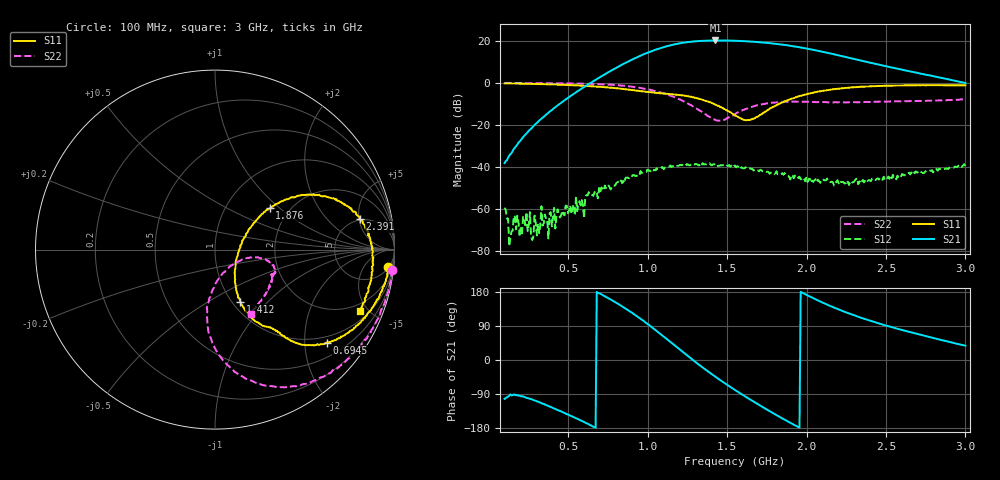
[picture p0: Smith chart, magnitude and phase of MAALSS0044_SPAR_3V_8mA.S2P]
!Part No: MAALSS0044
!Bias: Vdd=3V, Idd=8mA (R1=open)
!2-port de-embedded S-parameters
!Date: Wed Sep 14 16:43:49 2011
!Temp: +25c
!REF Task A17L_2309
!Fixture: 25050XX Rev00
!Test System: Agilent Technologies,E5071C,MY46106711,A.09.61
!Data & Calibration Information:
!Freq	S11:SOLT2(ON)	S21:SOLT2(ON)	S12:SOLT2(ON)	S22:SOLT2(ON)
!PortZ  Port1:50+j0  Port2:50+j0
# Hz S dB R 50
!Freq(Hz)	S11(dB) 	S11(Angle)	S21(dB) 	S21(Angle)	S12(dB) 	S12(Angle)	S22(dB) 	S22(Angle)
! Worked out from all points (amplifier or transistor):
!   401 points, 100 MHz to 3 GHz, reference 50 ohm
!   highest |S21| = 20.3 dB at 1.427 GHz (marker M1)
!   |S21| within 3 dB of that: 1.108 GHz to 1.936 GHz (827.6 MHz wide, 54.4 % of centre)
!   unconditionally stable (mu >= 1): start of sweep to end of sweep
!   at 578.5 MHz: K = 10.84, MAG = 14.3 dB, |S12| = -58.4 dB
!   at 1.55 GHz: K = 4.32, MAG = 20.4 dB, |S12| = -39.3 dB
!   at 3 GHz: K = 8.99, MAG = 7.2 dB, |S12| = -39.6 dB
!   S11 on the Smith chart (normalised r, x): 100 MHz: 6, -19; 694.5 MHz: 0.84, -2.52; 1.412 GHz: 1.09, -0.71; 1.876 GHz: 1.59, +0.86; 2.391 GHz: 4.83, +5.12; 3 GHz: 1.49, -4.42
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1e8  -0.27 -5.6  -38.19 -102.5  -59.46 101.5  -0.04 -6.5
1.3625e8  -0.27 -8.0  -33.97 -90.6  -74.02 111.5  -0.07 -8.9
5.8575e8  -1.28 -33.7  -2.65 -160.7  -55.86 167.7  -0.36 -39.3
6.945e8  -1.83 -39.8  2.52 176.2  -50.10 164.8  -0.59 -48.4
8.105e8  -2.60 -45.8  7.54 149.1  -47.35 137.3  -1.06 -59.4
9.1925e8  -3.54 -50.1  11.75 119.5  -44.25 138.1  -1.95 -70.7
9.9175e8  -4.20 -51.5  14.21 97.5  -42.48 118.4  -2.89 -78.5
1.0715e9  -4.90 -52.9  16.41 72.1  -40.86 108.2  -4.35 -86.6
1.16575e9  -5.50 -54.6  18.35 40.2  -39.47 90.3  -6.68 -94.4
1.26e9  -6.39 -59.1  19.56 8.2  -39.29 71.8  -10.08 -97.5
1.3325e9  -7.77 -62.6  20.02 -15.3  -38.57 58.1  -13.40 -91.8
1.41225e9  -9.78 -64.1  20.24 -39.7  -38.75 39.9  -17.28 -70.2
1.42675e9  -10.34 -63.5  20.27 -44.1  -39.52 38.8  -17.62 -63.5
1.55e9  -15.57 -48.9  20.12 -79.1  -39.34 16.0  -14.80 -15.3
1.62975e9  -17.68 -13.2  19.84 -100.3  -40.37 -0.5  -12.12 -10.5
1.724e9  -14.51 24.0  19.29 -124.1  -42.09 -12.6  -10.10 -13.0
1.87625e9  -8.37 37.1  17.98 -160.7  -44.26 -51.4  -9.02 -19.0
2.03575e9  -4.78 31.8  15.91 164.7  -46.59 -92.3  -9.05 -23.4
2.18075e9  -2.92 23.4  13.48 136.9  -48.15 -109.3  -9.15 -23.3
2.391e9  -1.68 11.9  9.83 105.0  -46.36 -161.3  -9.02 -25.3
2.5215e9  -1.32 5.2  7.61 88.2  -45.68 -167.2  -8.89 -29.9
3e9  -1.14 -23.1  -0.04 37.9  -39.55 -174.6  -7.76 -60.7
